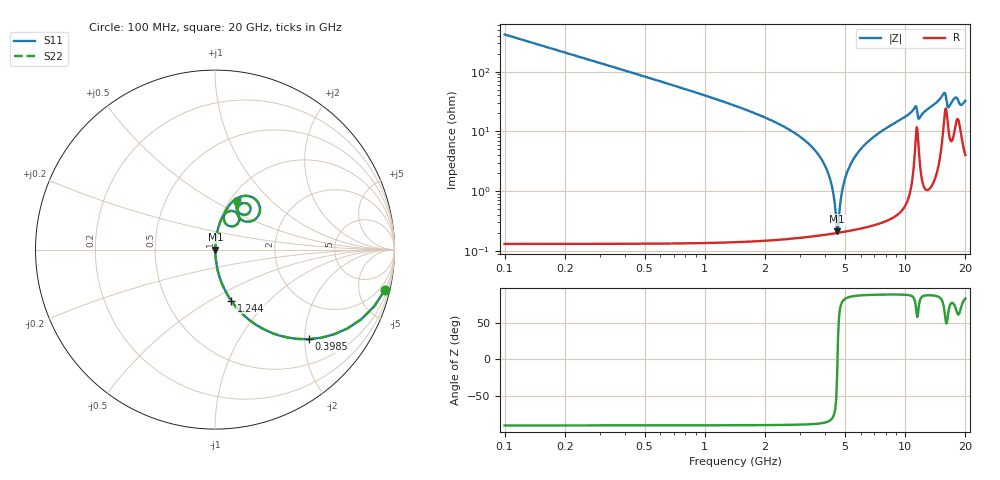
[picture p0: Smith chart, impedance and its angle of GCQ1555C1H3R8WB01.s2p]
!Murata Part Number: GCQ1555C1H3R8WB01
!These Parameters are Measured in Series Mode Connection
!Data Generated on Mar 13, 2026
!  o--ll--o
!Port1  Port2
!  o------o
!Operation Temp=25[degC], DC Bias Voltage=0[V]
!Freq. Start=100[MHz] Stop=20[GHz] 401[Steps]
# Hz S RI R 50
!Freq.(Hz) S11(Real) S11(Imag) S21(Real) S21(Imag) S12(Real) S12(Imag) S22(Real) S22(Imag)
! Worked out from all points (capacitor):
!   401 points, 100 MHz to 20 GHz, reference 50 ohm
!   read as one part in series: C = 3.8 pF near 199.5 MHz
!   lowest |Z| = 213 mohm at 4.577 GHz (marker M1)
!   series resonance near 4.597 GHz, so ESL is about 320 pH
!   S11 on the Smith chart (normalised r, x): 100 MHz: 1.00, -8.37; 398.5 MHz: 1.00, -2.09; 1.244 GHz: 1.00, -0.62; 20 GHz: 1.08, +0.64
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1e8  0.946 -0.2259  0.054 0.2259  0.054 0.2259  0.946 -0.2259
3.985e8  0.5211 -0.4989  0.4789 0.4989  0.4789 0.4989  0.5211 -0.4989
7.4675e8  0.2303 -0.4198  0.7697 0.4198  0.7697 0.4198  0.2303 -0.4198
1.24425e9  0.0898 -0.2837  0.9102 0.2837  0.9102 0.2837  0.0898 -0.2837
3.43325e9  0.00465 -0.0539  0.9954 0.0539  0.9954 0.0539  0.00465 -0.0539
4.1795e9  0.0022 -0.0174  0.9978 0.0174  0.9978 0.0174  0.0022 -0.0174
4.32875e9  0.00205 -0.011  0.998 0.011  0.998 0.011  0.00205 -0.011
4.5775e9  0.00198 -0.000758  0.998 0.000758  0.998 0.000758  0.00198 -0.000758
4.677e9  0.00202 0.00319  0.998 -0.00319  0.998 -0.00319  0.00202 0.00319
4.92575e9  0.00223 0.0127  0.9978 -0.0127  0.9978 -0.0127  0.00223 0.0127
5.274e9  0.0028 0.0254  0.9972 -0.0254  0.9972 -0.0254  0.0028 0.0254
6.7665e9  0.00805 0.0736  0.992 -0.0736  0.992 -0.0736  0.00805 0.0736
1.005e10  0.0356 0.1697  0.9644 -0.1697  0.9644 -0.1697  0.0356 0.1697
1.1244e10  0.1057 0.2132  0.8943 -0.2132  0.8943 -0.2132  0.1057 0.2132
1.17415e10  0.0624 0.142  0.9376 -0.142  0.9376 -0.142  0.0624 0.142
1.338325e10  0.0701 0.234  0.9299 -0.234  0.9299 -0.234  0.0701 0.234
1.557225e10  0.216 0.2869  0.784 -0.2869  0.784 -0.2869  0.216 0.2869
1.63185e10  0.1536 0.1624  0.8464 -0.1624  0.8464 -0.1624  0.1536 0.1624
1.67165e10  0.1223 0.2115  0.8777 -0.2115  0.8777 -0.2115  0.1223 0.2115
1.77115e10  0.1774 0.257  0.8226 -0.257  0.8226 -0.257  0.1774 0.257
1.89055e10  0.1405 0.2009  0.8595 -0.2009  0.8595 -0.2009  0.1405 0.2009
2e10  0.1222 0.271  0.8778 -0.271  0.8778 -0.271  0.1222 0.271
